PROGRAM Communication
VAR
	fbMBUSKL6781	:	FB_MBUSKL6781;
END_VAR

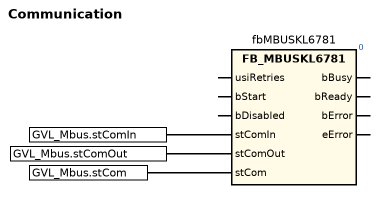
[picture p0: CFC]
fbMBUSKL6781(stComIn := GVL_Mbus.stComIn, stComOut := GVL_Mbus.stComOut, stCom := GVL_Mbus.stCom); // FB_MBUSKL6781

END_PROGRAM
